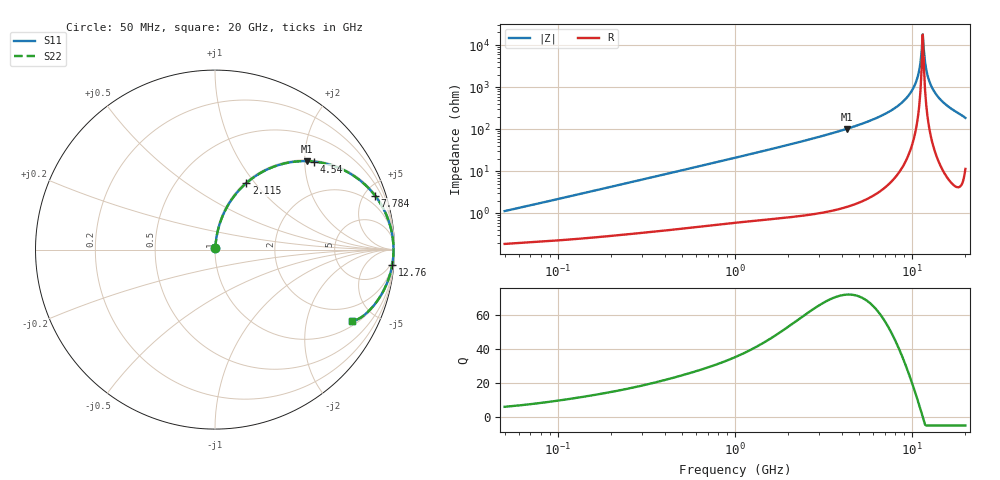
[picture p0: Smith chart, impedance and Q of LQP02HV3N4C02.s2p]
!Murata Part Number: LQP02HV3N4C02
!These Parameters are Measured in Series Mode Connection
!  o--[Z]--o
!Port1  Port2
!  o-------o
!Freq. Start=50[MHz] Stop=20[GHz], 401[Steps]
# Hz S RI R 50
!Freq.(Hz) S11(Real) S11(Imag) S21(Real) S21(Imag) S12(Real) S12(Imag) S22(Real) S22(Imag)
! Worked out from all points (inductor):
!   401 points, 50 MHz to 20 GHz, reference 50 ohm
!   read as one part in series: L = 3.53 nH near 51.52 MHz
!   highest Q = 71.8 at 4.276 GHz (marker M1), where L = 3.81 nH
!   self-resonance near 11.49 GHz
!   S11 on the Smith chart (normalised r, x): 50 MHz: 1.00, +0.02; 2.115 GHz: 1.02, +0.90; 4.54 GHz: 1.03, +2.22; 7.784 GHz: 1.12, +5.91; 12.76 GHz: 2, -22; 20 GHz: 1.23, -3.72
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5e7  0.00201 0.0112  0.998 -0.0112  0.998 -0.0112  0.00201 0.0112
1.364002e8  0.00339 0.0294  0.9966 -0.0294  0.9966 -0.0294  0.00339 0.0294
3.721004e8  0.00989 0.0778  0.9901 -0.0778  0.9901 -0.0778  0.00989 0.0778
1e9  0.0474 0.1987  0.9526 -0.1987  0.9526 -0.1987  0.0474 0.1987
2.114743e9  0.1744 0.3704  0.8256 -0.3704  0.8256 -0.3704  0.1744 0.3704
2.728004e9  0.2658 0.4339  0.7342 -0.4339  0.7342 -0.4339  0.2658 0.4339
4.275624e9  0.511 0.493  0.489 -0.493  0.489 -0.493  0.511 0.493
4.539627e9  0.5505 0.4905  0.4495 -0.4905  0.4495 -0.4905  0.5505 0.4905
7.442007e9  0.8694 0.3274  0.1306 -0.3274  0.1306 -0.3274  0.8694 0.3274
7.784049e9  0.8924 0.2996  0.1076 -0.2996  0.1076 -0.2996  0.8924 0.2996
9.041845e9  0.9541 0.1945  0.0459 -0.1945  0.0459 -0.1945  0.9541 0.1945
1.004137e10  0.9813 0.112  0.0187 -0.112  0.0187 -0.112  0.9813 0.112
1.066139e10  0.9903 0.0629  0.00973 -0.0629  0.00973 -0.0629  0.9903 0.0629
1.098561e10  0.9929 0.038  0.00711 -0.038  0.00711 -0.038  0.9929 0.038
1.115139e10  0.9937 0.0254  0.00627 -0.0254  0.00627 -0.0254  0.9937 0.0254
1.149051e10  0.9945 0.000358  0.00555 -0.000358  0.00555 -0.000358  0.9945 0.000358
1.166392e10  0.9943 -0.0122  0.00566 0.0122  0.00566 0.0122  0.9943 -0.0122
1.220001e10  0.9921 -0.0498  0.00793 0.0498  0.00793 0.0498  0.9921 -0.0498
1.276073e10  0.9869 -0.0872  0.0131 0.0872  0.0131 0.0872  0.9869 -0.0872
1.375312e10  0.9721 -0.1482  0.0279 0.1482  0.0279 0.1482  0.9721 -0.1482
1.504638e10  0.9443 -0.2182  0.0557 0.2182  0.0557 0.2182  0.9443 -0.2182
2e10  0.7633 -0.3955  0.2367 0.3955  0.2367 0.3955  0.7633 -0.3955
